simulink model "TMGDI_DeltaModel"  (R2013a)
settings: Solver=ode45  StartTime=0  StopTime=0.4  FixedStep=1e-4
PreLoadFcn:
  | warning('off','sm:sli:setup:compile:LocalSolverNotSupported')
InitFcn:
  |  SimParam.IC = SM2_InitCondConstrFnc(RawParam,IC);
model workspace (MAT data in the model file):
  handle : class17 (value not decoded)
  handle : class17 (value not decoded)
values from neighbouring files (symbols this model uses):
  RawParam = RobotParamGather(ParamLib)    [TMGDI_main.m]    (also in DeltaModelMain_v2.m; main_TimeSimulation.m; MGI.m = y)
libraries: SM2_BallJointPartsLib x6, SM2_ForeArmPartsLib x6, SM2_MotorPartsLib x3, SM2_ArmPartsLib x3, SM2_FramePartsLib x1, ElecDriverLib x1, SM2_ToolPartsLib x1

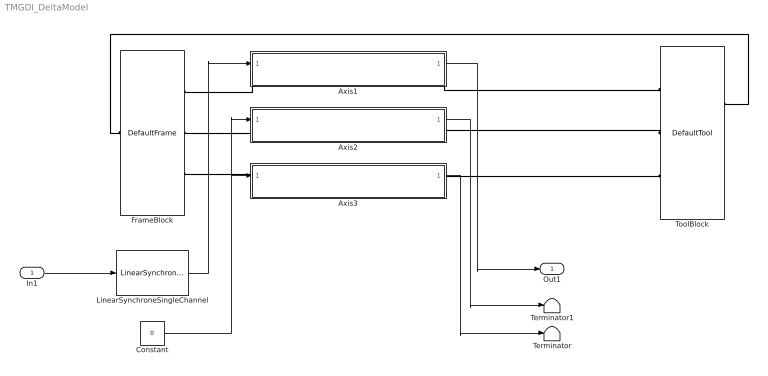
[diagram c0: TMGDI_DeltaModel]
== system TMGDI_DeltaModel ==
  In1 : Inport
  Axis1 : Subsystem
  Axis2 : Subsystem
  Axis3 : Subsystem
  Constant : Constant  Value=0
  FrameBlock : SM2_FramePartsLib/DefaultFrame
  LinearSynchroneSingleChannel : ElecDriverLib/LinearSynchroneSingleChannel  VariantControl=driverVarLinearSynchrone
  Terminator : Terminator
  Terminator1 : Terminator
  ToolBlock : SM2_ToolPartsLib/DefaultTool
  Out1 : Outport
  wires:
  Axis1/1(Alpha) -> Out1/1
  Axis2/1(Alpha) -> Terminator1/1
  Axis3/1(Alpha) -> Terminator/1
  LinearSynchroneSingleChannel/1 -> Axis1/1(Torque)
  In1/1 -> LinearSynchroneSingleChannel/1
  Constant/1 -> Axis2/1(Torque), Axis3/1(Torque)
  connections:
  Axis1/LConn1 -- FrameBlock/RConn1
  Axis2/LConn1 -- FrameBlock/RConn2
  Axis3/LConn1 -- FrameBlock/RConn3
  FrameBlock/LConn1 -- ToolBlock/LConn1
  Axis1/RConn1 -- ToolBlock/RConn1
  ToolBlock/RConn2 -- Axis2/RConn1
  Axis3/RConn1 -- ToolBlock/RConn3

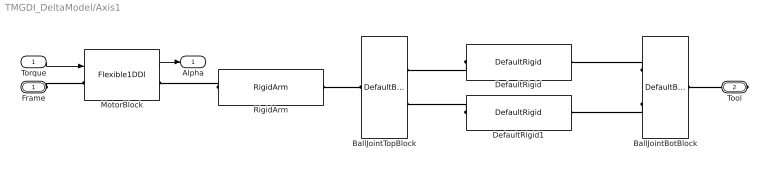
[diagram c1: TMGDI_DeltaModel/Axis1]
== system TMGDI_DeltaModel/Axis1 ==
  Torque : Inport
  BallJointBotBlock : SM2_BallJointPartsLib/DefaultBallJointBotPair
  BallJointTopBlock : SM2_BallJointPartsLib/DefaultBallJointTopPair
  DefaultRigid : SM2_ForeArmPartsLib/DefaultRigid  VariantControl=foreArmVarDefault
  DefaultRigid1 : SM2_ForeArmPartsLib/DefaultRigid  VariantControl=foreArmVarDefault
  MotorBlock : SM2_MotorPartsLib/Flexible1DDl  VariantControl=motorVarFlex1
  RigidArm : SM2_ArmPartsLib/RigidArm  VariantControl=armVarDefault
  Frame : PMIOPort  Port=1  Side=Left
  Tool : PMIOPort  Port=2  Side=Right
  Alpha : Outport
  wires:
  Torque/1 -> MotorBlock/1
  MotorBlock/1 -> Alpha/1
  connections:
  RigidArm/LConn1 -- MotorBlock/RConn1
  Frame/RConn1 -- MotorBlock/LConn1
  RigidArm/RConn1 -- BallJointTopBlock/RConn1
  Tool/RConn1 -- BallJointBotBlock/RConn1
  DefaultRigid1/LConn1 -- BallJointTopBlock/LConn2
  DefaultRigid/LConn1 -- BallJointTopBlock/LConn1
  BallJointBotBlock/LConn1 -- DefaultRigid/RConn1
  BallJointBotBlock/LConn2 -- DefaultRigid1/RConn1

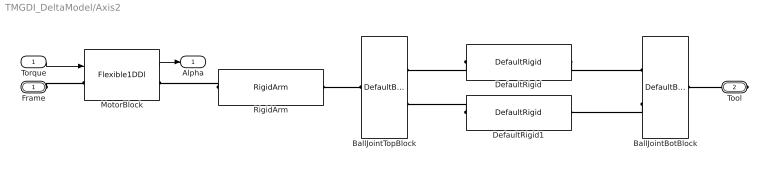
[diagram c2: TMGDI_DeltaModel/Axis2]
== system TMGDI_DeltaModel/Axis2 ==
  Torque : Inport
  BallJointBotBlock : SM2_BallJointPartsLib/DefaultBallJointBotPair
  BallJointTopBlock : SM2_BallJointPartsLib/DefaultBallJointTopPair
  DefaultRigid : SM2_ForeArmPartsLib/DefaultRigid  VariantControl=foreArmVarDefault
  DefaultRigid1 : SM2_ForeArmPartsLib/DefaultRigid  VariantControl=foreArmVarDefault
  MotorBlock : SM2_MotorPartsLib/Flexible1DDl  VariantControl=motorVarFlex1
  RigidArm : SM2_ArmPartsLib/RigidArm  VariantControl=armVarDefault
  Frame : PMIOPort  Port=1  Side=Left
  Tool : PMIOPort  Port=2  Side=Right
  Alpha : Outport
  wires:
  Torque/1 -> MotorBlock/1
  MotorBlock/1 -> Alpha/1
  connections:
  RigidArm/LConn1 -- MotorBlock/RConn1
  Frame/RConn1 -- MotorBlock/LConn1
  RigidArm/RConn1 -- BallJointTopBlock/RConn1
  Tool/RConn1 -- BallJointBotBlock/RConn1
  DefaultRigid1/LConn1 -- BallJointTopBlock/LConn2
  DefaultRigid/LConn1 -- BallJointTopBlock/LConn1
  DefaultRigid/RConn1 -- BallJointBotBlock/LConn1
  BallJointBotBlock/LConn2 -- DefaultRigid1/RConn1

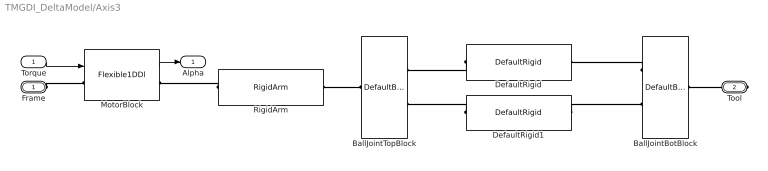
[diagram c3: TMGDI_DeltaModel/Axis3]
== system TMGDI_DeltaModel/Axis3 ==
  Torque : Inport
  BallJointBotBlock : SM2_BallJointPartsLib/DefaultBallJointBotPair
  BallJointTopBlock : SM2_BallJointPartsLib/DefaultBallJointTopPair
  DefaultRigid : SM2_ForeArmPartsLib/DefaultRigid  VariantControl=foreArmVarDefault
  DefaultRigid1 : SM2_ForeArmPartsLib/DefaultRigid  VariantControl=foreArmVarDefault
  MotorBlock : SM2_MotorPartsLib/Flexible1DDl  VariantControl=motorVarFlex1
  RigidArm : SM2_ArmPartsLib/RigidArm  VariantControl=armVarDefault
  Frame : PMIOPort  Port=1  Side=Left
  Tool : PMIOPort  Port=2  Side=Right
  Alpha : Outport
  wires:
  Torque/1 -> MotorBlock/1
  MotorBlock/1 -> Alpha/1
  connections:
  RigidArm/LConn1 -- MotorBlock/RConn1
  Frame/RConn1 -- MotorBlock/LConn1
  RigidArm/RConn1 -- BallJointTopBlock/RConn1
  Tool/RConn1 -- BallJointBotBlock/RConn1
  DefaultRigid1/LConn1 -- BallJointTopBlock/LConn2
  DefaultRigid/LConn1 -- BallJointTopBlock/LConn1
  DefaultRigid1/RConn1 -- BallJointBotBlock/LConn2
  BallJointBotBlock/LConn1 -- DefaultRigid/RConn1
